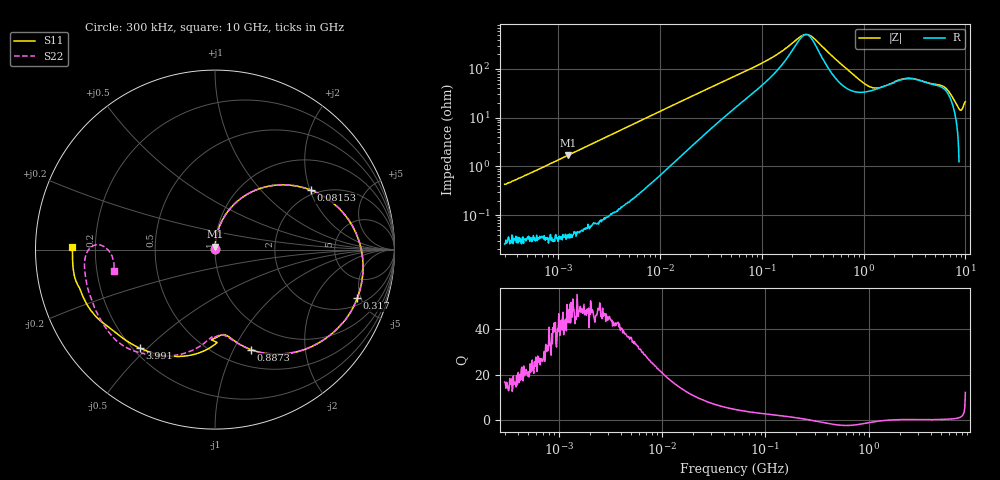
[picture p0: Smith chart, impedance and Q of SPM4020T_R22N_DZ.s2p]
! S-Parameter Data Generated by TDK Corporation
! Copyright(C) 2024 TDK Corporation.
! All Rights Reserved.
! TDK P/N: SPM4020T-R22N-DZ (SMD / SMT Inductor (Coil))
! Property: L=220nH at 100kHz
! Size(LxWxT): 4.3x4.1x2mm
! Model Type: s2p (Touchstone File Format Version 1.0)
! Frequency: DC=Yes Start=0.3MHz Stop=10000MHz 802points Log-sweep
! Model Generated on May 28, 2024
! Terms and conditions regarding TDK Simulation Models:
! 1)This simulation model is being provided solely for informational
!  purposes. Please refer to the specifications of the products in
!  terms of detailed characteristics of such products.
! 2)In no event shall TDK Corporation of any of its subsidiaries be
!  liable for any loss or damage arising, directly or indirectly,
!  from any information contained in this simulation model, including,
!  but not limited to loss or damages arising from any inaccuracies,
!  omissions or errors in connection with such information.
! 3)Any and all copyrights on this simulation model are owned by
!  TDK Corporation.  Duplication or redistribution of this simulation
!  model without prior written permission from TDK Corporation
!  is prohibited.
! 4)This simulation model is subject to any modification or change
!  without any prior notice.
! 5)Neither TDK Corporation nor any of its subsidiaries shall make any
!  warranty, express or implied, including but not limited to the
!  correctness, implied warranties of merchantability and fitness for
!  a particular purpose with respect to this simulation models.
! 6)The use of this simulation model shall be deemed to have consented
!  to the terms and conditions hereof.
! Port Assignments:
!  1 ---@@@--- 2
! Applicable Conditions:
!  Temperature = 25 degC
!  DC Bias Current = 0 A
!  Small Signal Operation
# Hz S MA R 50
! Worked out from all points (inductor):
!   801 points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, 300 kHz to 10 GHz, reference 50 ohm
!   read as one part in series: L = 220 nH near 318.3 kHz
!   highest Q = 48.3 at 1.254 MHz (marker M1), where L = 216 nH
!   self-resonance near 271.8 MHz
!   S11 on the Smith chart (normalised r, x): 300 kHz: 1.00, +0.01; 81.53 MHz: 1.84, +2.02; 317 MHz: 2.56, -4.65; 887.3 MHz: 0.68, -1.17; 3.991 GHz: 0.23, -0.48; 10 GHz: 0.11, +0.01
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300000  0.004843 89.2  0.9995 -0.2  0.9993 -0.2  0.004778 92.9
1254421  0.0167 88.1  0.9995 -1.0  0.9993 -1.0  0.01668 88.2
1713600  0.02266 87.6  0.9992 -1.4  0.9991 -1.4  0.02268 87.7
9671944  0.1248 79.7  0.9861 -7.6  0.9863 -7.6  0.1248 79.7
2.441527e7  0.2926 65.5  0.9234 -17.9  0.9235 -17.9  0.2926 65.5
5.477226e7  0.5179 44.2  0.7451 -32.6  0.7451 -32.6  0.5179 44.2
8.153051e7  0.6273 32.0  0.6093 -40.1  0.6094 -40.1  0.6274 32.1
1.405283e8  0.7532 14.2  0.3913 -47.5  0.3914 -47.5  0.7533 14.3
2.53844e8  0.8335 -8.7  0.1689 -21.0  0.169 -21.0  0.8339 -8.4
3.126428e8  0.8379 -18.2  0.179 10.6  0.179 10.6  0.8383 -17.8
3.169586e8  0.8376 -18.9  0.1826 12.2  0.1826 12.2  0.8381 -18.5
5.414944e8  0.7582 -46.1  0.4274 23.2  0.4274 23.2  0.7595 -45.6
6.821612e8  0.6863 -58.2  0.5292 13.1  0.5292 13.1  0.6881 -57.7
8.872678e8  0.5915 -70.3  0.6055 -1.8  0.6056 -1.8  0.5944 -69.9
1.212691e9  0.5004 -80.0  0.624 -21.6  0.6241 -21.6  0.5038 -80.2
1.767019e9  0.4843 -87.9  0.5481 -46.0  0.5481 -46.0  0.4813 -88.6
2.477118e9  0.5713 -96.8  0.4374 -63.4  0.4374 -63.4  0.5345 -97.7
3.991169e9  0.6903 -127.2  0.3184 -86.4  0.3184 -86.4  0.6929 -122.2
6.172341e9  0.7394 -145.4  0.2318 -113.4  0.2319 -113.4  0.7491 -141.1
8.09931e9  0.784 -163.5  0.1682 -139.5  0.1681 -139.6  0.7374 -167.9
9.217363e9  0.7973 -172.6  0.1275 -150.2  0.1277 -150.1  0.6794 178.2
1e10  0.7947 178.9  0.1088 -144.3  0.1088 -144.5  0.5749 -168.2
